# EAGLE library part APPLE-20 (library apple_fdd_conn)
Apple Disk II connector
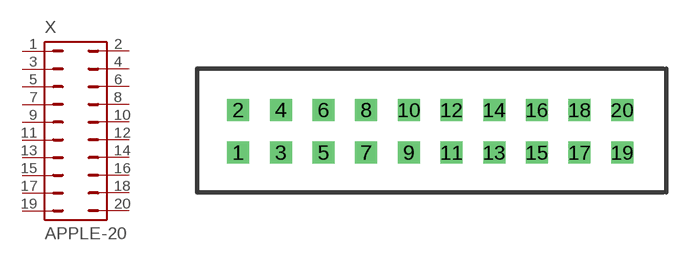
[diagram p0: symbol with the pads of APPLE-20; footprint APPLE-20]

Designator prefix X

## APPLE-20  [APPLE-20]
1  1  pas
2  2  pas
3  3  pas
4  4  pas
5  5  pas
6  6  pas
7  7  pas
8  8  pas
9  9  pas
10  10  pas
11  11  pas
12  12  pas
13  13  pas
14  14  pas
15  15  pas
16  16  pas
17  17  pas
18  18  pas
19  19  pas
20  20  pas

## Footprint APPLE-20 (pad centres in mm)
Apple Disk II connector
drill 0.8 square: 1 -11.43,-1.27; 2 -11.43,1.27; 3 -8.89,-1.27; 4 -8.89,1.27; 5 -6.35,-1.27; 6 -6.35,1.27; 7 -3.81,-1.27; 8 -3.81,1.27; 9 -1.27,-1.27; 10 -1.27,1.27; 11 1.27,-1.27; 12 1.27,1.27; 13 3.81,-1.27; 14 3.81,1.27; 15 6.35,-1.27; 16 6.35,1.27; 17 8.89,-1.27; 18 8.89,1.27; 19 11.43,-1.27; 20 11.43,1.27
